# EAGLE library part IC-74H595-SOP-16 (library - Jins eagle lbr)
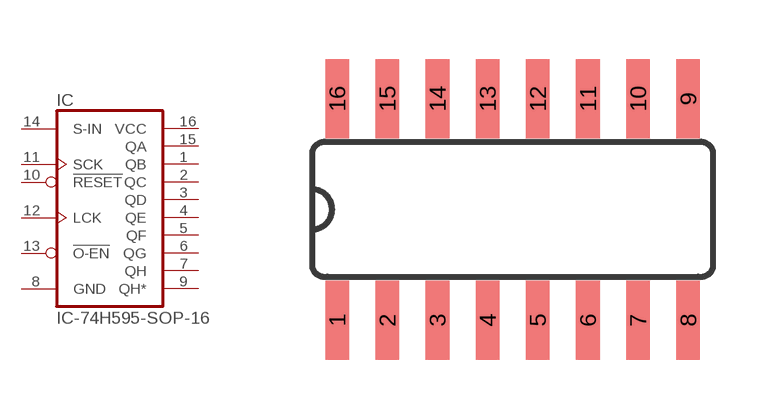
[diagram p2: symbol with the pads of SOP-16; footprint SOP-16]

Designator prefix IC

## IC-74H595-SOP-16  [SOP-16]
1  QB  hiz
2  QC  hiz
3  QD  hiz
4  QE  hiz
5  QF  hiz
6  QG  hiz
7  QH  hiz
8  GND  pwr
9  QH*  hiz
10  !RESET  in
11  SCK  in
12  LCK  in
13  !O-EN  in
14  S-IN  in
15  QA  hiz
16  VCC  pwr

## Footprint SOP-16 (pad centres in mm)
smd 0.6 x 2: 1 -3.945,-2.76; 2 -2.675,-2.76; 3 -1.405,-2.76; 4 -0.135,-2.76; 5 1.135,-2.76; 6 2.405,-2.76; 7 3.675,-2.76; 8 4.945,-2.76; 9 4.945,2.84; 10 3.675,2.84; 11 2.405,2.84; 12 1.135,2.84; 13 -0.135,2.84; 14 -1.405,2.84; 15 -2.675,2.84; 16 -3.945,2.84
